| TEXAS INSTRUMENTS INCORPORATED
| Standard Linear and Logic Group
| IBIS Model of SN74LV4066A
| QUADRUPLE BILATERAL ANALOG SWITCHES
| This file contains package information for the following:
|  TSSOP 14-pin (PW) package as [Component] LV4066A_PW
|  SOP 14-pin (NS) package as [Component] LV4066A_NS
|  PDIP 14-pin (N) package as [Component] LV4066A_N
|  TVSOP 14-pin (DGV) package as [Component] LV4066A_DGV
|  SSOP 14-pin (DB) package as [Component] LV4066A_DB
|  SOIC 14-pin (D) package as [Component] LV4066A_D
|  QFN 14-pin (RGY) package as [Component] LV4066A_RGY
| This device can be powered at the following Vccs:
|  2.5 volt Vcc
|  3.3 volt Vcc
|  5 volt Vcc
| This file provides unique models under the [Model Selector] for each Vcc.
| For operation at a specific Vcc, select the appropriate model after each
| [Model Selector] keyword.
[IBIS Ver]   3.2
[Comment char]  |_char
[File Name]   sn74lv4066a.ibs
[File Rev]   1.1 | h_die
[Date]   March 19, 2003
[Source]   Data created from TI-SPICE simulations at TI-SLL.
[Notes]   The following is an IBIS list for the LV4066A.
   Please contact sllibis@ti.com with questions and
   comments concerning SLL IBIS models.
   This IBIS model is created from a BA (back annotated
   netlist).
   - Power-clamp data has been deleted from the input model
   since there is no power-clamp diode.
   - C_comp values are taken at a different test condition than
   the Ci/Cio in data sheet.
   - Non-monotonic data due to device characteristics.
[Disclaimer] Property of Texas Instruments Incorporated.  Unauthorized
   reproduction and/or distribution is strictly prohibited.
   This product is protected under copyright law.
   Created  2003, (C) Copyright  2003, Texas Instruments
   Incorporated, All Rights Reserved
   UNLESS THERE IS A SIGNED, WRITTEN AGREEMENT TO THE
   CONTRARY, TEXAS INSTRUMENTS (TI) IS PROVIDING THE IBIS
   MODELS  AND WITHOUT ANY WARRANTY, EXPRESSED OR
   IMPLIED.  TI assumes no liability for:
   1) the accuracy of the IBIS models provided to your
   company;
   2) the proper functioning of these IBIS Models in your
   design or for any resulting applications; or
   3) infringement of patents, copyrights or intellectual
   property rights resulting from your use of these IBIS
   models.
   TI provides IBIS Models as a service to our customers.
   You and your company shall not distribute, sell or give
   these models to anyone else without prior written
   permission from TI.
   TI reserves the right to make changes to our products or
   to discontinue any semiconductor product or service
   without notice, and advises our customers to obtain the
   latest version of relevant information to verify, before
   placing orders, that the information being relied on is
   current.
   Please be aware that your receipt and use of the IBIS
   information provided shall serve as acceptance of these
   terms and conditions.  If you do not accept these terms,
   you should return or destroy the IBIS models and any
   other accompanying information immediately.
| Component LV4066A_PW 14-pin TSSOP
[Component]   LV4066A_PW
[Manufacturer]   Texas Instruments, Inc.
[Package]
|   typ   min   max
R_pkg   3.200e-02   2.900e-02   3.500e-02
L_pkg   2.378e-09   2.170e-09   2.680e-09
C_pkg   3.140e-13   2.700e-13   3.350e-13
[Pin]   signal_name   model_name   R_pin   L_pin   C_pin
1   1A   LV4066A_IO   3.300e-02   2.618e-09   3.300e-13
2   1B   LV4066A_IO   3.100e-02   2.313e-09   3.170e-13
3   2B   LV4066A_IO   3.000e-02   2.310e-09   3.140e-13
4   2A   LV4066A_IO   3.100e-02   2.173e-09   2.720e-13
5   2C   LV4066A_IN   3.000e-02   2.204e-09   3.090e-13
6   3C   LV4066A_IN   3.200e-02   2.315e-09   3.170e-13
7   GND   GND   3.500e-02   2.680e-09   3.350e-13
8   3A   LV4066A_IO   3.300e-02   2.640e-09   3.330e-13
9   3B   LV4066A_IO   3.400e-02   2.347e-09   3.190e-13
10   4B   LV4066A_IO   2.900e-02   2.277e-09   3.130e-13
11   4A   LV4066A_IO   3.100e-02   2.170e-09   2.700e-13
12   4C   LV4066A_IN   3.100e-02   2.244e-09   3.110e-13
13   1C   LV4066A_IN   3.300e-02   2.343e-09   3.210e-13
14   VCC   POWER   3.500e-02   2.657e-09   3.320e-13
| Component LV4066A_NS 14-pin SOP
[Component]   LV4066A_NS
[Manufacturer]   Texas Instruments, Inc.
[Package]
|   typ   min   max
R_pkg   4.500e-02   3.900e-02   5.400e-02
L_pkg   3.796e-09   2.561e-09   4.952e-09
C_pkg   5.280e-13   2.880e-13   7.100e-13
[Pin]   signal_name   model_name   R_pin   L_pin   C_pin
1   1A   LV4066A_IO   4.700e-02   4.867e-09   7.060e-13
2   1B   LV4066A_IO   5.100e-02   4.083e-09   5.920e-13
3   2B   LV4066A_IO   4.100e-02   2.915e-09   3.760e-13
4   2A   LV4066A_IO   3.900e-02   2.561e-09   2.880e-13
5   2C   LV4066A_IN   4.100e-02   3.101e-09   4.300e-13
6   3C   LV4066A_IN   4.700e-02   4.047e-09   5.890e-13
7   GND   GND   5.100e-02   4.909e-09   7.000e-13
8   3A   LV4066A_IO   4.500e-02   4.784e-09   6.940e-13
9   3B   LV4066A_IO   5.400e-02   4.176e-09   5.970e-13
10   4B   LV4066A_IO   3.900e-02   3.287e-09   4.490e-13
11   4A   LV4066A_IO   3.900e-02   2.586e-09   2.940e-13
12   4C   LV4066A_IN   4.000e-02   2.802e-09   3.710e-13
13   1C   LV4066A_IN   4.900e-02   4.080e-09   5.930e-13
14   VCC   POWER   5.200e-02   4.952e-09   7.100e-13
| Component LV4066A_N 14-pin PDIP
[Component]   LV4066A_N
[Manufacturer]   Texas Instruments, Inc.
[Package]
|   typ   min   max
R_pkg   4.500e-02   3.700e-02   6.300e-02
L_pkg   5.407e-09   3.922e-09   6.942e-09
C_pkg   3.890e-13   2.050e-13   6.040e-13
[Pin]   signal_name   model_name   R_pin   L_pin   C_pin
1   1A   LV4066A_IO   6.300e-02   6.942e-09   6.040e-13
2   1B   LV4066A_IO   3.700e-02   6.200e-09   4.060e-13
3   2B   LV4066A_IO   4.200e-02   4.389e-09   3.220e-13
4   2A   LV4066A_IO   3.800e-02   3.922e-09   2.050e-13
5   2C   LV4066A_IN   3.900e-02   4.301e-09   2.980e-13
6   3C   LV4066A_IN   3.800e-02   5.329e-09   3.560e-13
7   GND   GND   5.300e-02   6.510e-09   5.440e-13
8   3A   LV4066A_IO   5.300e-02   6.437e-09   5.390e-13
9   3B   LV4066A_IO   3.900e-02   5.352e-09   3.470e-13
10   4B   LV4066A_IO   4.200e-02   4.473e-09   2.970e-13
11   4A   LV4066A_IO   4.400e-02   4.326e-09   2.250e-13
12   4C   LV4066A_IN   4.200e-02   4.295e-09   2.800e-13
13   1C   LV4066A_IN   4.200e-02   6.318e-09   4.180e-13
14   VCC   POWER   6.100e-02   6.900e-09   6.030e-13
| Component LV4066A_DGV 14-pin TVSOP
[Component]   LV4066A_DGV
[Manufacturer]   Texas Instruments, Inc.
[Package]
|   typ   min   max
R_pkg   3.500e-02   2.000e-02   4.500e-02
L_pkg   2.499e-09   2.077e-09   2.966e-09
C_pkg   3.610e-13   3.050e-13   4.160e-13
[Pin]   signal_name   model_name   R_pin   L_pin   C_pin
1   1A   LV4066A_IO   2.700e-02   2.717e-09   3.730e-13
2   1B   LV4066A_IO   3.700e-02   2.434e-09   3.980e-13
3   2B   LV4066A_IO   3.400e-02   2.200e-09   3.160e-13
4   2A   LV4066A_IO   2.000e-02   2.077e-09   3.090e-13
5   2C   LV4066A_IN   3.000e-02   2.147e-09   3.050e-13
6   3C   LV4066A_IN   4.200e-02   2.580e-09   4.080e-13
7   GND   GND   3.900e-02   2.921e-09   3.850e-13
8   3A   LV4066A_IO   3.300e-02   2.841e-09   3.800e-13
9   3B   LV4066A_IO   4.200e-02   2.611e-09   4.100e-13
10   4B   LV4066A_IO   3.800e-02   2.331e-09   3.290e-13
11   4A   LV4066A_IO   2.600e-02   2.223e-09   3.190e-13
12   4C   LV4066A_IN   3.400e-02   2.259e-09   3.130e-13
13   1C   LV4066A_IN   4.500e-02   2.681e-09   4.160e-13
14   VCC   POWER   4.200e-02   2.966e-09   3.860e-13
| Component LV4066A_DB 14-pin SSOP
[Component]   LV4066A_DB
[Manufacturer]   Texas Instruments, Inc.
[Package]
|   typ   min   max
R_pkg   4.400e-02   4.100e-02   4.600e-02
L_pkg   3.551e-09   3.258e-09   3.927e-09
C_pkg   4.020e-13   3.600e-13   4.210e-13
[Pin]   signal_name   model_name   R_pin   L_pin   C_pin
1   1A   LV4066A_IO   4.600e-02   3.927e-09   4.080e-13
2   1B   LV4066A_IO   4.400e-02   3.587e-09   4.210e-13
3   2B   LV4066A_IO   4.100e-02   3.289e-09   3.980e-13
4   2A   LV4066A_IO   4.200e-02   3.258e-09   3.600e-13
5   2C   LV4066A_IN   4.100e-02   3.286e-09   4.030e-13
6   3C   LV4066A_IN   4.400e-02   3.586e-09   4.210e-13
7   GND   GND   4.600e-02   3.927e-09   4.080e-13
8   3A   LV4066A_IO   4.600e-02   3.927e-09   4.080e-13
9   3B   LV4066A_IO   4.400e-02   3.586e-09   4.210e-13
10   4B   LV4066A_IO   4.100e-02   3.286e-09   4.030e-13
11   4A   LV4066A_IO   4.300e-02   3.258e-09   3.600e-13
12   4C   LV4066A_IN   4.100e-02   3.289e-09   3.980e-13
13   1C   LV4066A_IN   4.400e-02   3.587e-09   4.210e-13
14   VCC   POWER   4.600e-02   3.927e-09   4.080e-13
| Component LV4066A_D 14-pin SOIC
[Component]   LV4066A_D
[Manufacturer]   Texas Instruments, Inc.
[Package]
|   typ   min   max
R_pkg   3.100e-02   2.800e-02   3.400e-02
L_pkg   3.109e-09   2.462e-09   3.889e-09
C_pkg   4.730e-13   3.630e-13   6.280e-13
[Pin]   signal_name   model_name   R_pin   L_pin   C_pin
1   1A   LV4066A_IO   3.300e-02   3.854e-09   6.220e-13
2   1B   LV4066A_IO   3.200e-02   3.188e-09   4.730e-13
3   2B   LV4066A_IO   2.800e-02   2.462e-09   3.770e-13
4   2A   LV4066A_IO   3.100e-02   2.596e-09   3.630e-13
5   2C   LV4066A_IN   2.800e-02   2.521e-09   3.720e-13
6   3C   LV4066A_IN   3.400e-02   3.250e-09   4.760e-13
7   GND   GND   3.400e-02   3.889e-09   6.280e-13
8   3A   LV4066A_IO   3.400e-02   3.889e-09   6.280e-13
9   3B   LV4066A_IO   3.400e-02   3.250e-09   4.760e-13
10   4B   LV4066A_IO   2.800e-02   2.521e-09   3.720e-13
11   4A   LV4066A_IO   3.100e-02   2.596e-09   3.640e-13
12   4C   LV4066A_IN   2.800e-02   2.462e-09   3.770e-13
13   1C   LV4066A_IN   3.200e-02   3.188e-09   4.730e-13
14   VCC   POWER   3.300e-02   3.854e-09   6.220e-13
| Component LV4066A_RGY 14-pin QFN
[Component]   LV4066A_RGY
[Manufacturer]   Texas Instruments, Inc.
[Package]
|   typ   min   max
R_pkg   2.900e-02   2.300e-02   4.100e-02
L_pkg   7.730e-10   6.570e-10   9.980e-10
C_pkg   1.360e-13   1.150e-13   1.560e-13
[Pin]   signal_name   model_name   R_pin   L_pin   C_pin
1   1A   LV4066A_IO   2.700e-02   8.310e-10   1.300e-13
2   1B   LV4066A_IO   2.700e-02   8.660e-10   1.350e-13
3   2B   LV4066A_IO   4.100e-02   9.980e-10   1.560e-13
4   2A   LV4066A_IO   3.100e-02   7.670e-10   1.420e-13
5   2C   LV4066A_IN   3.100e-02   7.650e-10   1.420e-13
6   3C   LV4066A_IN   3.100e-02   7.830e-10   1.440e-13
7   GND   GND   3.100e-02   7.810e-10   1.370e-13
8   3A   LV4066A_IO   2.300e-02   6.570e-10   1.150e-13
9   3B   LV4066A_IO   2.300e-02   8.140e-10   1.290e-13
10   4B   LV4066A_IO   2.800e-02   7.040e-10   1.290e-13
11   4A   LV4066A_IO   2.700e-02   6.720e-10   1.360e-13
12   4C   LV4066A_IN   2.700e-02   6.960e-10   1.380e-13
13   1C   LV4066A_IN   2.700e-02   7.250e-10   1.400e-13
14   VCC   POWER   3.000e-02   7.630e-10   1.360e-13
[Series Switch Groups]
| Function Group States
On  1 /   | 1A->1B 1C HIGH
On  2 /   | 2A->2B 2C HIGH
On  3 /   | 3A->3B 3C HIGH
On  4 /   | 4A->4B 4C HIGH
On  1 2 3 4 /   | Enable all
On  1 2 /   | Enable 1C Enable 2C
On  1 3 /   | Enable 1C Enable 3C
On  1 4 /   | Enable 1C Enable 4C
On  2 3 /   | Enable 2C Enable 3C
On  2 4 /   | Enable 2C Enable 4C
On  3 4 /   | Enable 3C Enable 4C
On  1 2 3 /   | Enable 1C Enable 2C Enable 3C
On  1 2 4 /   | Enable 1C Enable 2C Enable 4C
On  1 3 4 /   | Enable 1C Enable 3C Enable 4C
On  2 3 4 /   | Enable 2C Enable 3C Enable 4C
[Series Pin Mapping]   pin_2   model_name   function_table_group
1   2   LV4066A_IO_25_S   1
| 1   2   LV4066A_IO_33_S   1
| 1   2   LV4066A_IO_50_S   1
4   3   LV4066A_IO_25_S   2
| 4   3   LV4066A_IO_33_S   2
| 4   3   LV4066A_IO_50_S   2
8   9   LV4066A_IO_25_S   3
| 8   9   LV4066A_IO_33_S   3
| 8   9   LV4066A_IO_50_S   3
11   10   LV4066A_IO_25_S   4
| 11   10   LV4066A_IO_33_S   4
| 11   10   LV4066A_IO_50_S   4
| Model LV4066A_IN
[Model Selector]   LV4066A_IN
LV4066A_IN_25   2.5 volt Vcc
LV4066A_IN_33   3.3 volt Vcc
LV4066A_IN_50   5 volt Vcc
| Model LV4066A_IO
[Model Selector]   LV4066A_IO
LV4066A_IO_25   2.5 volt Vcc
LV4066A_IO_33   3.3 volt Vcc
LV4066A_IO_50   5 volt Vcc
| Model LV4066A_IO_S
[Model Selector]   LV4066A_IO_S
LV4066A_IO_25_S   2.5 volt Vcc
LV4066A_IO_33_S   3.3 volt Vcc
LV4066A_IO_50_S   5 volt Vcc
[Model]   LV4066A_IO_25_S
Model_type  Series_switch
| variable   typ   min   max
C_comp   0   0   0
[Temperature Range]   40   100   -40
| Ambient temperature   25   85   -40
[Voltage range]   2.5   2.3   2.7
[On]
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[Off]
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[Model]   LV4066A_IO_33_S
Model_type  Series_switch
| variable   typ   min   max
C_comp   0   0   0
[Temperature Range]   40   100   -40
| Ambient temperature   25   85   -40
[Voltage range]   3.3   3   3.6
[On]
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[Off]
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[Model]   LV4066A_IO_50_S
Model_type  Series_switch
| variable   typ   min   max
C_comp   0   0   0
[Temperature Range]   40   100   -40
| Ambient temperature   25   85   -40
[Voltage range]   5   4.5   5.5
[On]
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[Off]
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| Models and submodels in the file (9): LV4066A_IN_25 (Input), LV4066A_IN_33 (Input), LV4066A_IN_50 (Input), LV4066A_IO_25_S (Series_switch), LV4066A_IO_25 (Terminator), LV4066A_IO_33_S (Series_switch), LV4066A_IO_33 (Terminator), LV4066A_IO_50_S (Series_switch), LV4066A_IO_50 (Terminator)
